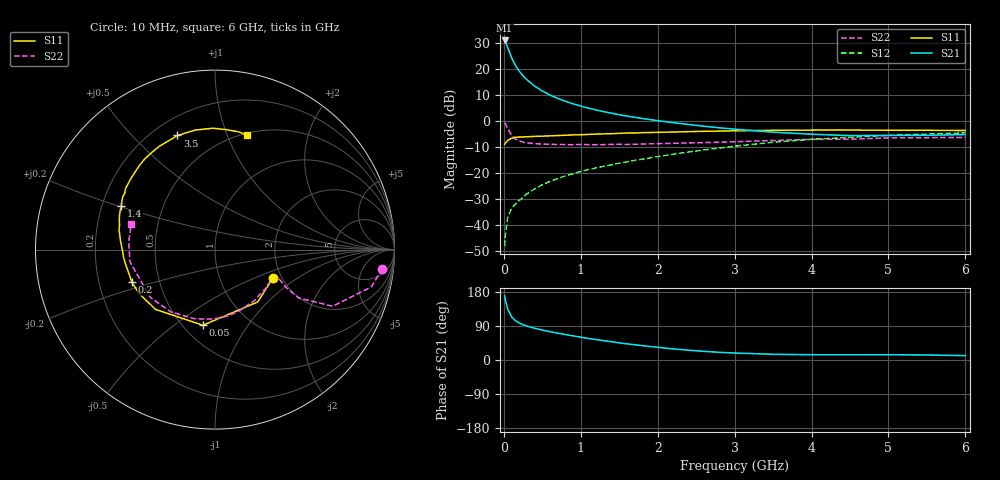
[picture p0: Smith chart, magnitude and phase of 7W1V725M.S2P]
! Infineon Technologies  Discrete & RF Semiconductors
! BFS17W
! Si NPN RF Bipolar Junction Transistor in SOT323
! VCE = 1.75 V  IC = 25 mA
! Common Emitter S-Parameters:  August  1999
# GHz  S  MA  R  50
!  f  S11  S21  S12  S22
! GHz  MAG  ANG  MAG  ANG  MAG  ANG  MAG  ANG
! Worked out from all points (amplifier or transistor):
!   36 points, 10 MHz to 6 GHz, reference 50 ohm
!   highest |S21| = 31.2 dB at 10 MHz (marker M1)
!   |S21| within 3 dB of that: start of sweep to 53.69 MHz
!   unconditionally stable (mu >= 1): 176.8 MHz to end of sweep
!   at 250 MHz: K = 1.18, MAG = 20.8 dB, |S12| = -29.4 dB
!   at 1.4 GHz: K = 1.31, MAG = 6.6 dB, |S12| = -16.8 dB
!   at 6 GHz: K = 1.11, MAG = -2.4 dB, |S12| = -4.5 dB
!   S11 on the Smith chart (normalised r, x): 10 MHz: 1.79, -0.66; 50 MHz: 0.62, -0.64; 200 MHz: 0.35, -0.17; 1.4 GHz: 0.28, +0.20; 3.5 GHz: 0.30, +0.68; 6 GHz: 0.52, +1.18
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0.01  0.3592 -26.6  36.14 169.1  0.0039 78.5  0.9385 -6.5
0.02  0.3764 -50.8  34.56 158.1  0.0063 73.3  0.8958 -13.4
0.05  0.4267 -99.1  26.44 134.2  0.014 62.3  0.7274 -25.7
0.1  0.4698 -134.8  16.89 114.1  0.0209 56.4  0.5392 -30.0
0.15  0.4891 -150.1  12.01 103.9  0.0255 57.4  0.4559 -28.3
0.2  0.4976 -158.8  9.266 97.7  0.0298 61.2  0.4181 -26.3
0.25  0.4975 -164.5  7.5 93.2  0.034 62.2  0.3948 -24.7
0.3  0.5022 -168.7  6.299 89.6  0.0398 65.0  0.3837 -24.0
0.4  0.5112 -174.9  4.765 83.7  0.0496 66.6  0.3684 -23.9
0.5  0.5154 -179.2  3.836 79.0  0.0597 68.4  0.3637 -24.7
0.6  0.5224 177.4  3.197 74.7  0.0694 69.2  0.3594 -26.2
0.7  0.5301 174.3  2.76 70.8  0.0789 69.9  0.3564 -28.4
0.9  0.5459 168.4  2.165 63.7  0.0972 70.3  0.3531 -33.6
1.1  0.5582 162.8  1.792 56.9  0.1172 70.3  0.3542 -39.8
1.4  0.5758 155.1  1.428 48.2  0.1447 70.0  0.3582 -49.9
1.8  0.6035 145.7  1.13 37.8  0.1856 69.5  0.363 -64.5
2.2  0.6197 136.3  0.941 29.4  0.2311 67.7  0.3757 -78.8
2.8  0.646 122.9  0.748 20.3  0.304 62.8  0.3936 -100.8
3.5  0.6692 108.2  0.616 15.1  0.3939 55.0  0.4256 -125.4
4.5  0.6763 91.0  0.529 13.9  0.4901 41.4  0.4503 -159.0
5.5  0.6692 78.8  0.536 13.2  0.5666 29.5  0.4831 174.6
6  0.6627 74.2  0.554 11.5  0.5971 23.8  0.4877 163.0
